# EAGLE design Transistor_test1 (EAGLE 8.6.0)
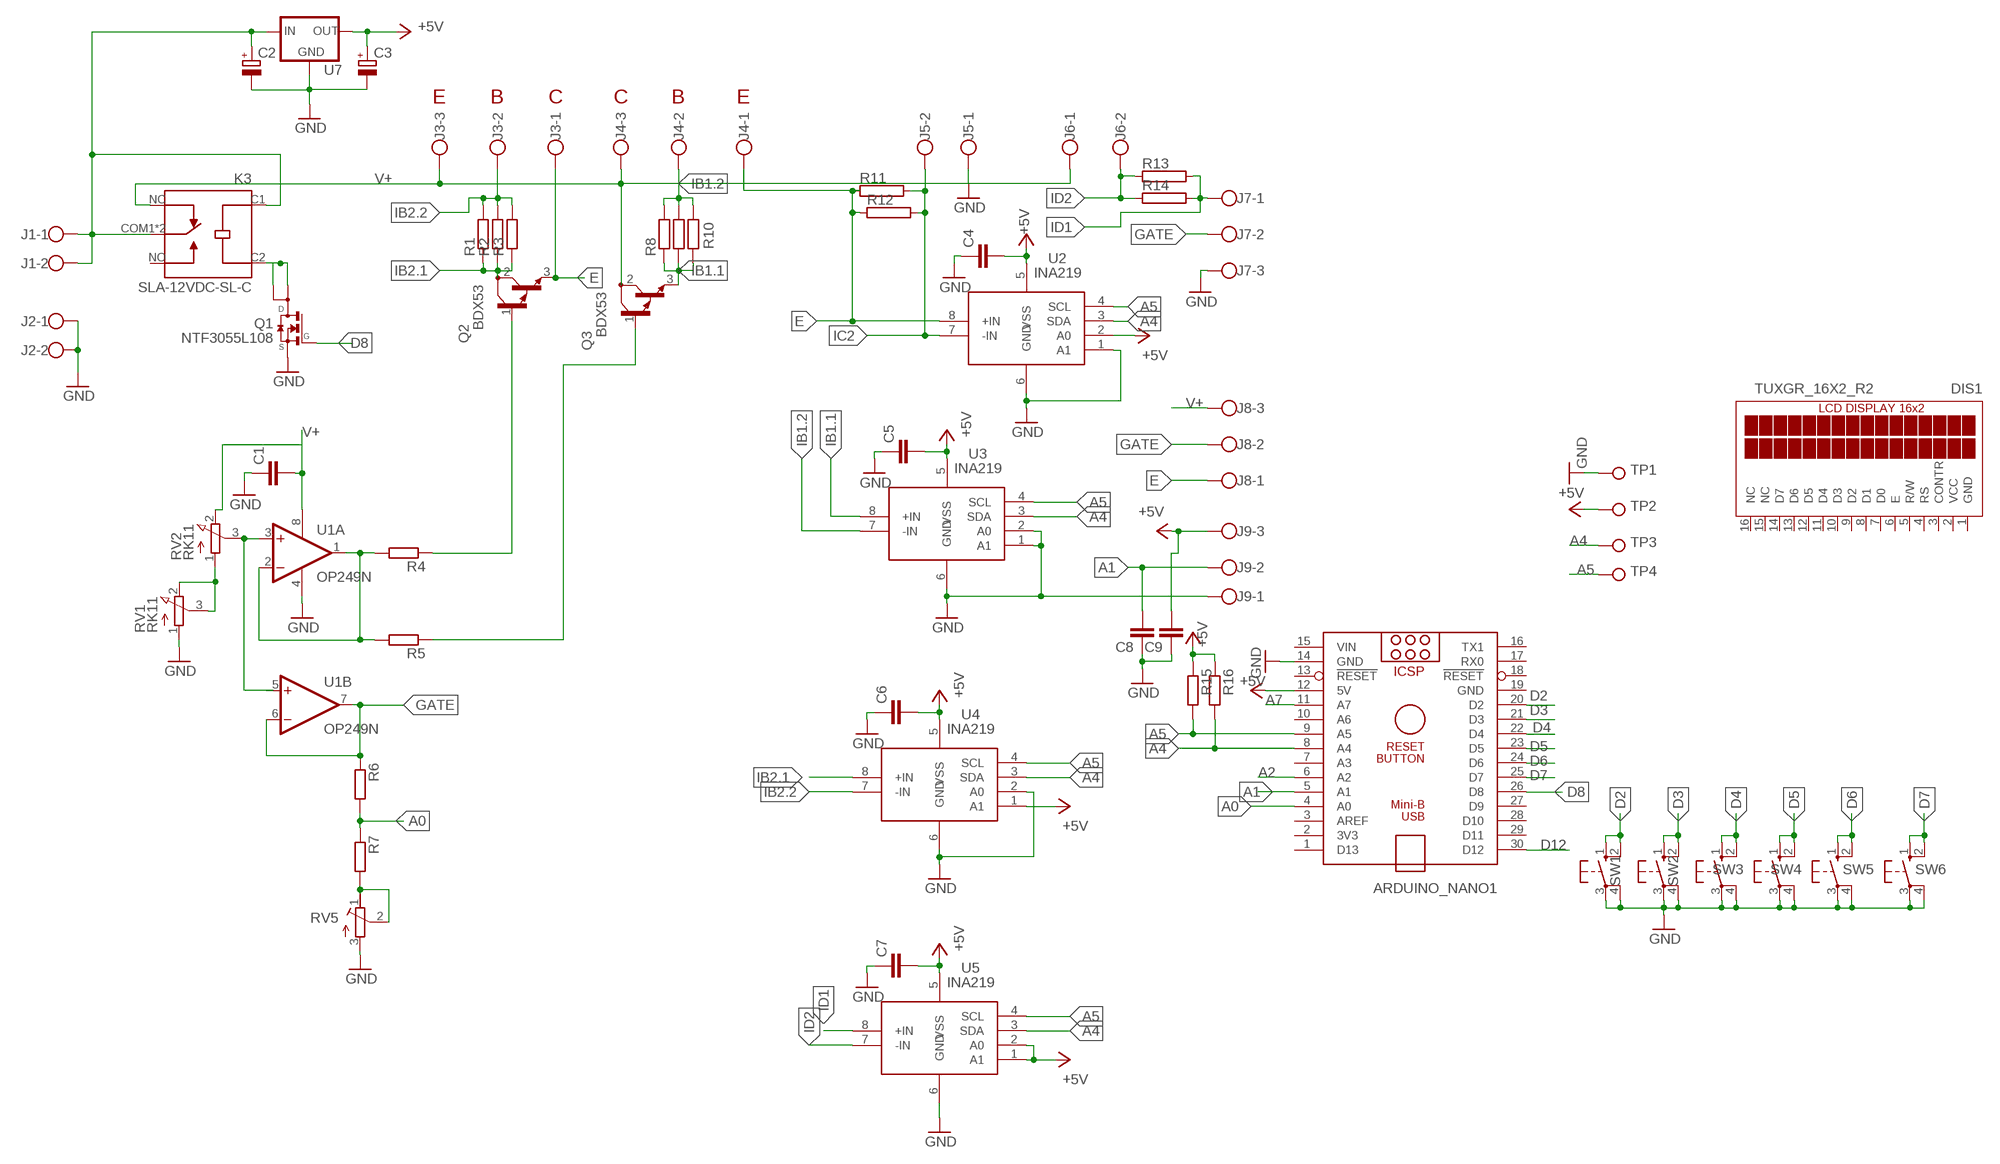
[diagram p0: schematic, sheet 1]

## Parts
ARDUINO_NANO1  ARDUINO_NANO  [ARDUINO_NANO]
C1  C-EUC1206  [C1206]
C2  CPOL-EUE2.5-7  [E2,5-7]
C3  CPOL-EUE2.5-7  [E2,5-7]
C4  C-EUC1206  [C1206]
C5  C-EUC1206  [C1206]
C6  C-EUC1206  [C1206]
C7  C-EUC1206  [C1206]
C8  C-EUC1206  [C1206]
C9  C-EUC1206  [C1206]
DIS1  TUXGR_16X2_R2  [TUXGR_16X2_R2]
J1  W237-102  [W237-102]
J2  W237-102  [W237-102]
J3  W237-103  [W237-103]
J4  W237-103  [W237-103]
J5  W237-102  [W237-102]
J6  W237-102  [W237-102]
J7  W237-103  [W237-103]
J8  W237-103  [W237-103]
J9  W237-103  [W237-103]
K3  SLA-12VDC-SL-C  [RELAY_SLA-12VDC-SL-C]
Q1  NTF3055L108  [SOT223]
Q2  BDX53  [TO220]
Q3  BDX53  [TO220]
R1  R-EU_R2512  [R2512]
R2  R-EU_R2512  [R2512]
R3  R-EU_R2512  [R2512]
R4  R-EU_R1206  [R1206]
R5  R-EU_R1206  [R1206]
R6  R-EU_R1206  [R1206]
R7  R-EU_R1206  [R1206]
R8  R-EU_R2512  [R2512]
R9  R-EU_R2512  [R2512]
R10  R-EU_R2512  [R2512]
R11  RAC07  [AC07]
R12  RAC07  [AC07]
R13  RAC07  [AC07]
R14  RAC07  [AC07]
R15  R-EU_R1206  [R1206]
R16  R-EU_R1206  [R1206]
RV1  RK11  PTV111  [PTV111]
RV2  RK11  PTV111  [PTV111]
RV5  R-TRIMM-3386-F  [R-TRIMM-3386F]
SW1  40-XX  [B3F-40XX]
SW2  40-XX  [B3F-40XX]
SW3  40-XX  [B3F-40XX]
SW4  40-XX  [B3F-40XX]
SW5  40-XX  [B3F-40XX]
SW6  40-XX  [B3F-40XX]
TP1  TPPAD1-13Y  [P1-13Y]
TP2  TPPAD1-13Y  [P1-13Y]
TP3  TPPAD1-13Y  [P1-13Y]
TP4  TPPAD1-13Y  [P1-13Y]
U1  OP249N  [DIL08]
U2  INA219  [SO08]
U3  INA219  [SO08]
U4  INA219  [SO08]
U5  INA219  [SO08]
U7  78MXXS  [78MXXS]

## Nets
+5V: ARDUINO_NANO1.12(5V) C3.+ C4.2 C5.2 C6.2 C7.2 C9.2 J9.3 R15.1 R16.1 TP2.TP U2.2(A0) U2.5(VSS) U3.5(VSS) U4.1(A1) U4.5(VSS) U5.1(A1) U5.2(A0) U5.5(VSS) U7.OUT
+15V: C2.+ J1.1 J1.2 K3.C1(COIL1) K3.COM1(COM) K3.COM2(COM) U7.IN
A0: ARDUINO_NANO1.4(A0) R6.2 R7.1
A1: ARDUINO_NANO1.5(A1) C8.2 J9.2
A2: ARDUINO_NANO1.6(A2)
A4: ARDUINO_NANO1.8(A4) R16.2 TP3.TP U2.3(SDA) U3.3(SDA) U4.3(SDA) U5.3(SDA)
A5: ARDUINO_NANO1.9(A5) R15.2 TP4.TP U2.4(SCL) U3.4(SCL) U4.4(SCL) U5.4(SCL)
A7: ARDUINO_NANO1.11(A7)
D2: ARDUINO_NANO1.20(D2) SW1.1(S) SW1.2(S1)
D3: ARDUINO_NANO1.21(D3) SW2.1(S) SW2.2(S1)
D4: ARDUINO_NANO1.22(D4) SW3.1(S) SW3.2(S1)
D5: ARDUINO_NANO1.23(D5) SW4.1(S) SW4.2(S1)
D6: ARDUINO_NANO1.24(D6) SW5.1(S) SW5.2(S1)
D7: ARDUINO_NANO1.25(D7) SW6.1(S) SW6.2(S1)
D8: ARDUINO_NANO1.26(D8) Q1.1(G)
D12: ARDUINO_NANO1.30(D12)
E: J3.1 J4.1 J8.1 Q2.3(E) R11.1 R12.1 U2.8(+IN)
GATE: J7.2 J8.2 R6.1 U1.6(B:-IN) U1.7(B:OUT)
GND: ARDUINO_NANO1.14(GND) C1.1 C2.- C3.- C4.1 C5.1 C6.1 C7.1 C8.1 C9.1 J2.1 J2.2 J5.1 J7.3 J9.1 Q1.3(S) RV1.1(A) RV5.3(E) SW1.3(P) SW1.4(P1) SW2.3(P) SW2.4(P1) SW3.3(P) SW3.4(P1) SW4.3(P) SW4.4(P1) SW5.3(P) SW5.4(P1) SW6.3(P) SW6.4(P1) TP1.TP U1.4(P:V-) U2.1(A1) U2.6(GND) U3.1(A1) U3.2(A0) U3.6(GND) U4.2(A0) U4.6(GND) U5.6(GND) U7.GND
IB1.1: Q3.3(E) R8.1 R9.1 R10.1 U3.8(+IN)
IB1.2: J4.2 R8.2 R9.2 R10.2 U3.7(-IN)
IB2.1: Q2.2(C) R1.1 R2.1 R3.1 U4.8(+IN)
IB2.2: J3.2 R1.2 R2.2 R3.2 U4.7(-IN)
IC2: J5.2 R11.2 R12.2 U2.7(-IN)
ID1: J7.1 R13.2 R14.2 U5.8(+IN)
ID2: J6.2 R13.1 R14.1 U5.7(-IN)
N$1: Q3.1(B) R5.1
N$2: R4.2 R5.2 U1.1(A:OUT) U1.2(A:-IN)
N$4: K3.C2(COIL2) Q1.2(D) Q1.4(D2)
N$5: RV1.2(E) RV1.3(S) RV2.1(A)
N$6: R7.2 RV5.1(A) RV5.2(S)
N$7: Q2.1(B) R4.1
N$11: RV2.3(S) U1.3(A:+IN) U1.5(B:+IN)
V+: C1.2 J3.3 J4.3 J6.1 J8.3 K3.NC Q3.2(C) RV2.2(E) U1.8(P:V+)
Unconnected: ARDUINO_NANO1.1(D13) ARDUINO_NANO1.2(3V3) ARDUINO_NANO1.3(AREF) ARDUINO_NANO1.7(A3) ARDUINO_NANO1.10(A6) ARDUINO_NANO1.13(!RESET) ARDUINO_NANO1.16(TX1) ARDUINO_NANO1.17(RX0) ARDUINO_NANO1.18(!RESET) ARDUINO_NANO1.27(D9) ARDUINO_NANO1.28(D10) ARDUINO_NANO1.29(D11) DIS1.3(CONTR) DIS1.4(RS) DIS1.5(R/W) DIS1.6(E) DIS1.7(D0) DIS1.8(D1) DIS1.9(D2) DIS1.10(D3) DIS1.11(D4) DIS1.12(D5) DIS1.13(D6) DIS1.14(D7) DIS1.15(NC) DIS1.16(NC) K3.NO

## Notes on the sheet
- E | B | C | C | B | E

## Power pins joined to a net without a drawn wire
GND: ARDUINO_NANO1.19(GND) DIS1.1(GND)
VCC: DIS1.2(VCC)
VIN: ARDUINO_NANO1.15(VIN)

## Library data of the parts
ARDUINO_NANO1 = ArduinoNanoV30:ARDUINO_NANO: Arduino Nano V3.0 Overview: The Arduino Nano is a small, complete, and breadboard-friendly board based on the ATmega328 (Arduino Nano 3.x) or ATmega168 (Arduino Nano 2.x). It has more or less the same functionality of the Arduino Duemilanove, but in a different package. It lacks only a DC power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
C1 C4-C9 = rcl:C-EU: CAPACITOR, European symbol
C2 C3 = rcl:CPOL-EU: POLARIZED CAPACITOR, European symbol
DIS1 = display-lcd:TUXGR_16X2_R2: Tuxgraphics LCD display 16x2 characters reflective, without background light Source: tuxgr_12x2_r2.pdf; OC_FARNELL: unknown; OC_NEWARK: unknown
J1 J2 J5 J6 = con-wago-500:W237-102: WAGO SCREW CLAMP; MPN: 237-102; OC_FARNELL: unknown; OC_NEWARK: 70K9898
J3 J4 J7-J9 = con-wago-500:W237-103: WAGO SCREW CLAMP; MPN: 237-103; OC_FARNELL: unknown; OC_NEWARK: 18M7116
K3 = SLA-12VDC-SL-C:SLA-12VDC-SL-C: SUBMINATURE HIGH POWER RELAY Check availability; AVAILABILITY: Not in stock; CHECK_PRICES: https://www.snapeda.com/parts/SLA-12VDC-SL-C/Songle+Relay/view-part/?ref=eda; DESCRIPTION: SUBMINATURE HIGH POWER RELAY; MF: Songle Relay; MP: SLA-12VDC-SL-C; PACKAGE: None; PRICE: None; SNAPEDA_LINK: https://www.snapeda.com/parts/SLA-12VDC-SL-C/Songle+Relay/view-part/?ref=snap
Q1 = NTF3055L108:NTF3055L108: N-Channel MOSFET 3.0 A, 60 V Check availability; AVAILABILITY: In Stock; CHECK_PRICES: https://www.snapeda.com/parts/NTF3055L108/Onsemi/view-part/?ref=eda; DESCRIPTION: N-Channel 60 V 3A (Ta) 1.3W (Ta) Surface Mount SOT-223 (TO-261); MF: ON Semiconductor; MP: NTF3055L108; PACKAGE: TO-261-4 ON Semiconductor; PRICE: None; PURCHASE-URL: https://www.snapeda.com/api/url_track_click_mouser/?unipart_id=2731930&manufacturer=ON Semiconductor&part_name=NTF3055L108&search_term=ntf3055; SNAPEDA_LINK: https://www.snapeda.com/parts/NTF3055L108/Onsemi/view-part/?ref=snap
Q2 Q3 = transistor:BDX53: NPN BIPOLAR DARLINGTON TRANSISTOR
R1-R3 R8-R10 = resistor:R-EU_: RESISTOR, European symbol
R4-R7 R15 R16 = rcl:R-EU_: RESISTOR, European symbol
R11-R14 = resistor-power:R: Power Resitor; OC_FARNELL: unknown; OC_NEWARK: unknown
RV1 RV2 = pot:PTV111
RV5 = rcl:R-TRIMM-3386-F
SW1-SW6 = switch-omron:40-XX: OMRON SWITCH; MF: OMRON COMPONENTS USA; MPN: B3F-4000; OC_FARNELL: 176434; OC_NEWARK: 36K3105
TP1-TP4 = testpad:TP: Test pad
U1 = linear:OP249: Dual, Precision JFET High Speed Operational Amplifier Source: http://www.analog.com/static/imported-files/data_sheets/OP249.pdf
U2-U5 = burr-brown:INA219: Bidirectional Current/Power Monitor With I2C Interface
U7 = v-reg:78MXXS: VOLTAGE REGULATOR

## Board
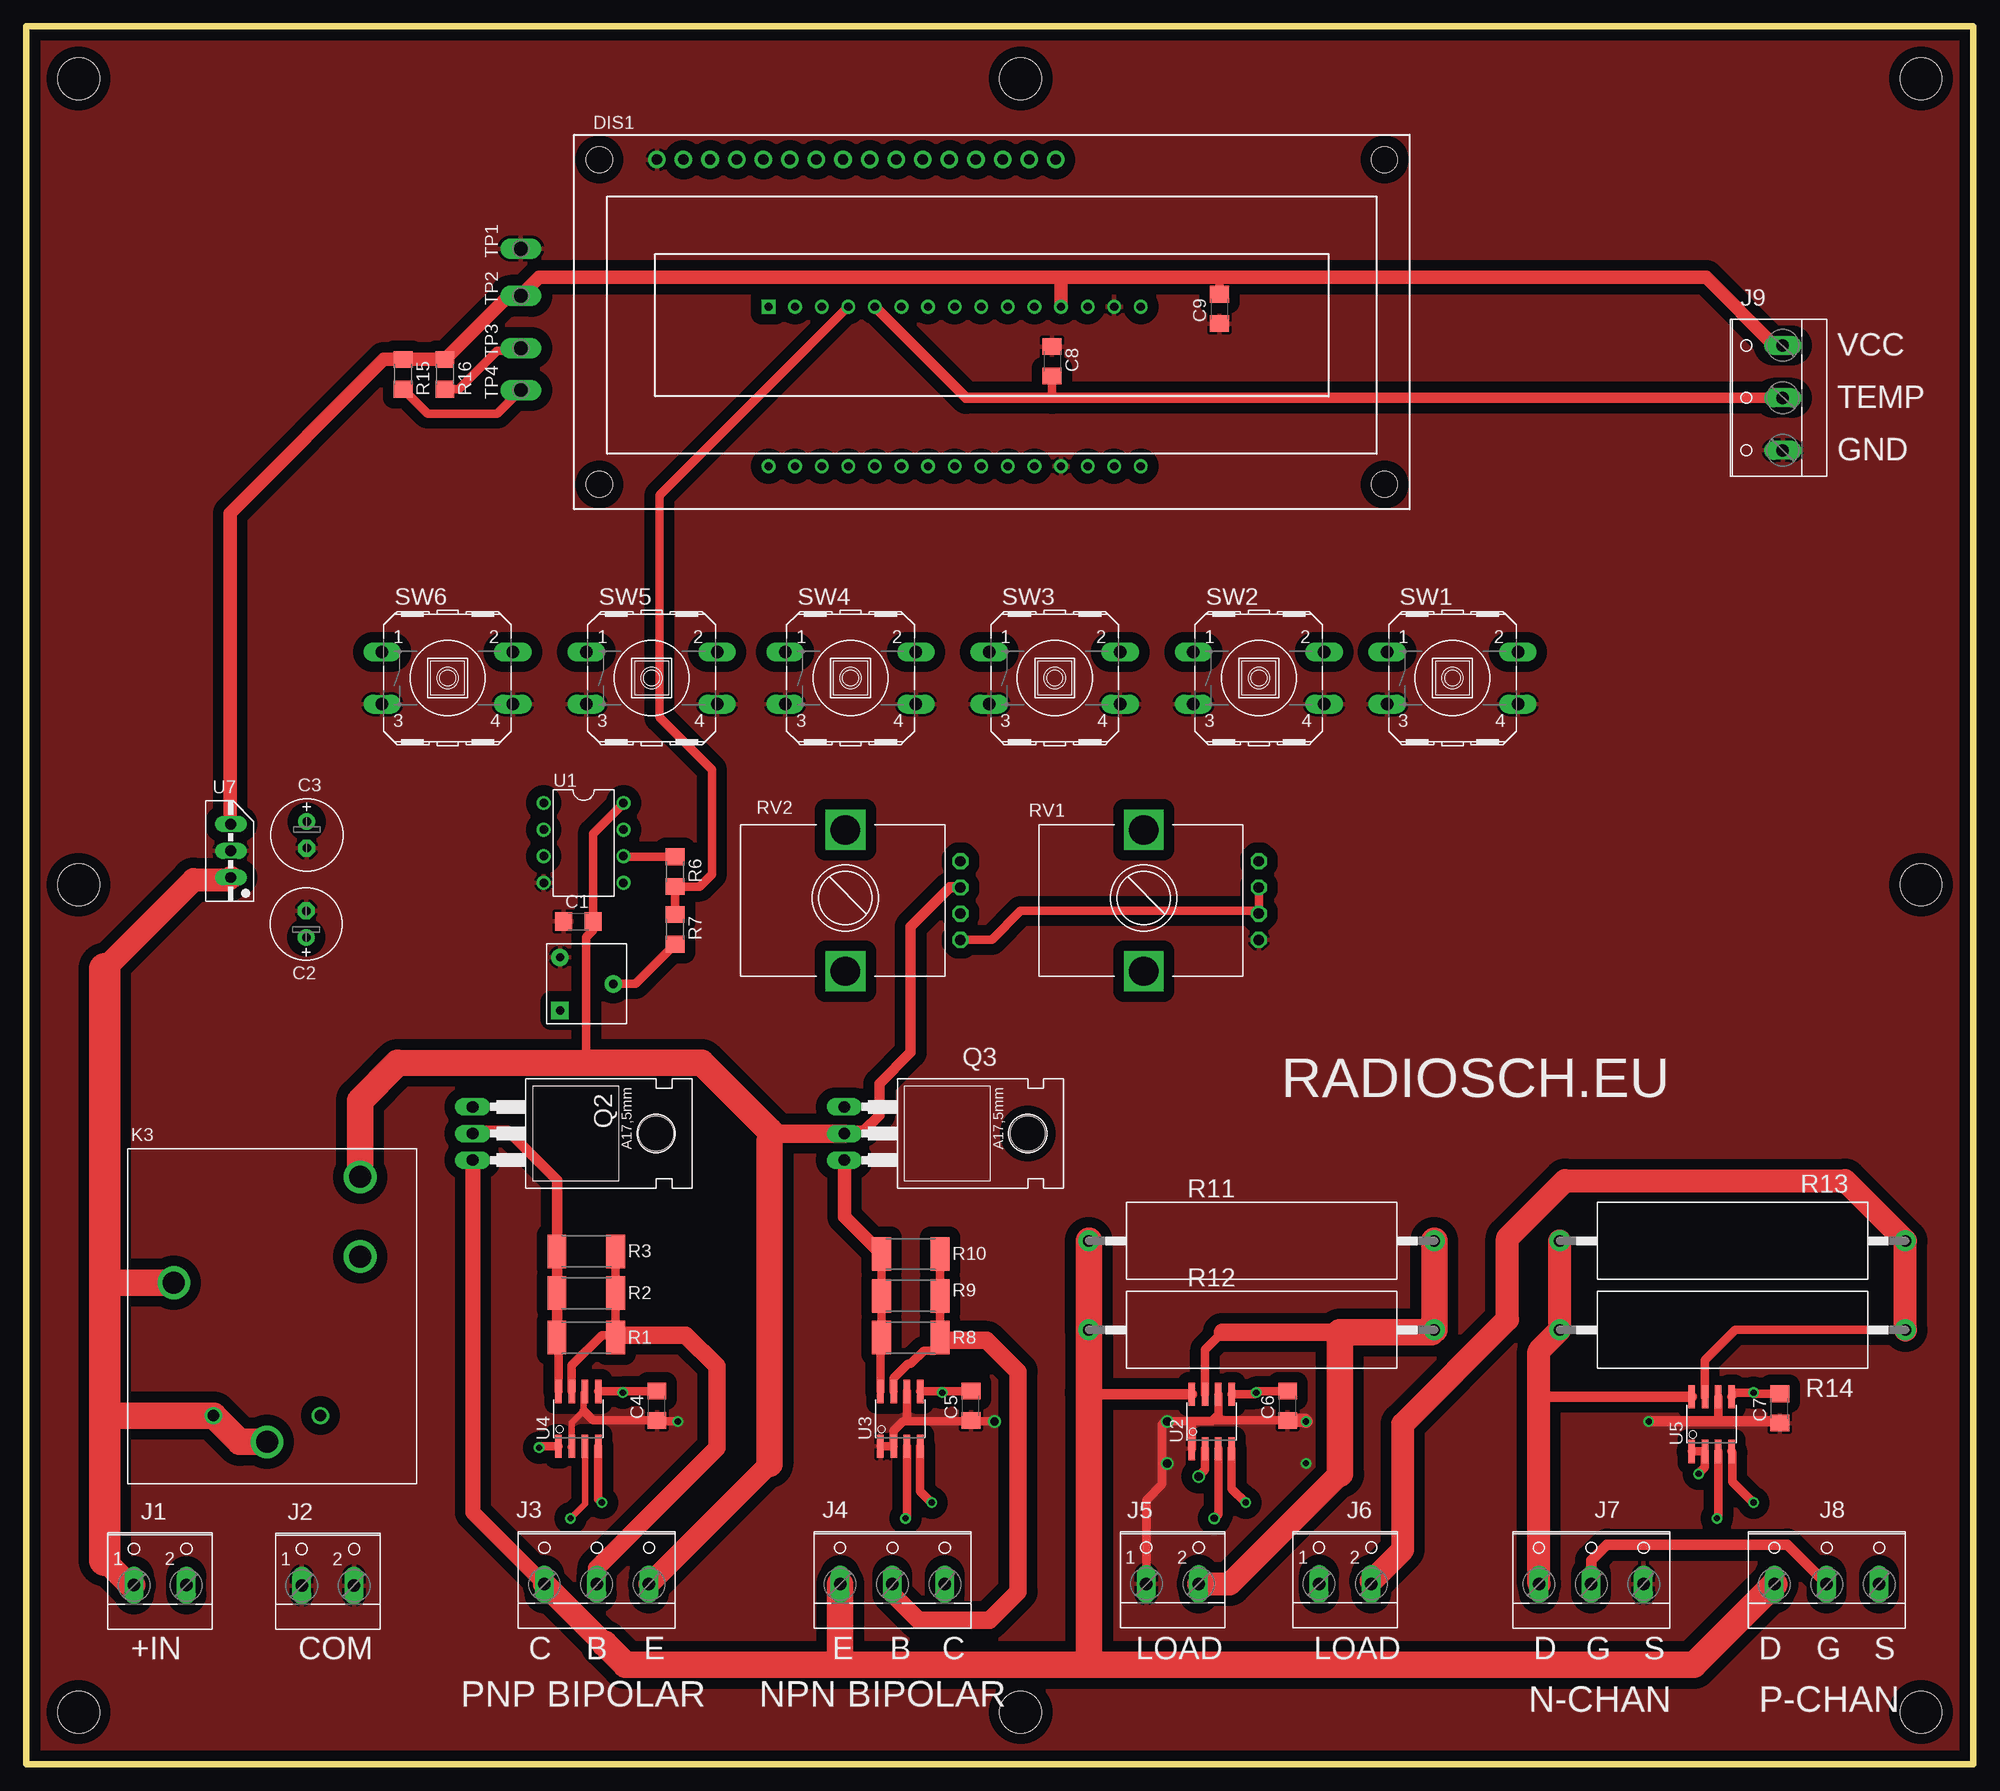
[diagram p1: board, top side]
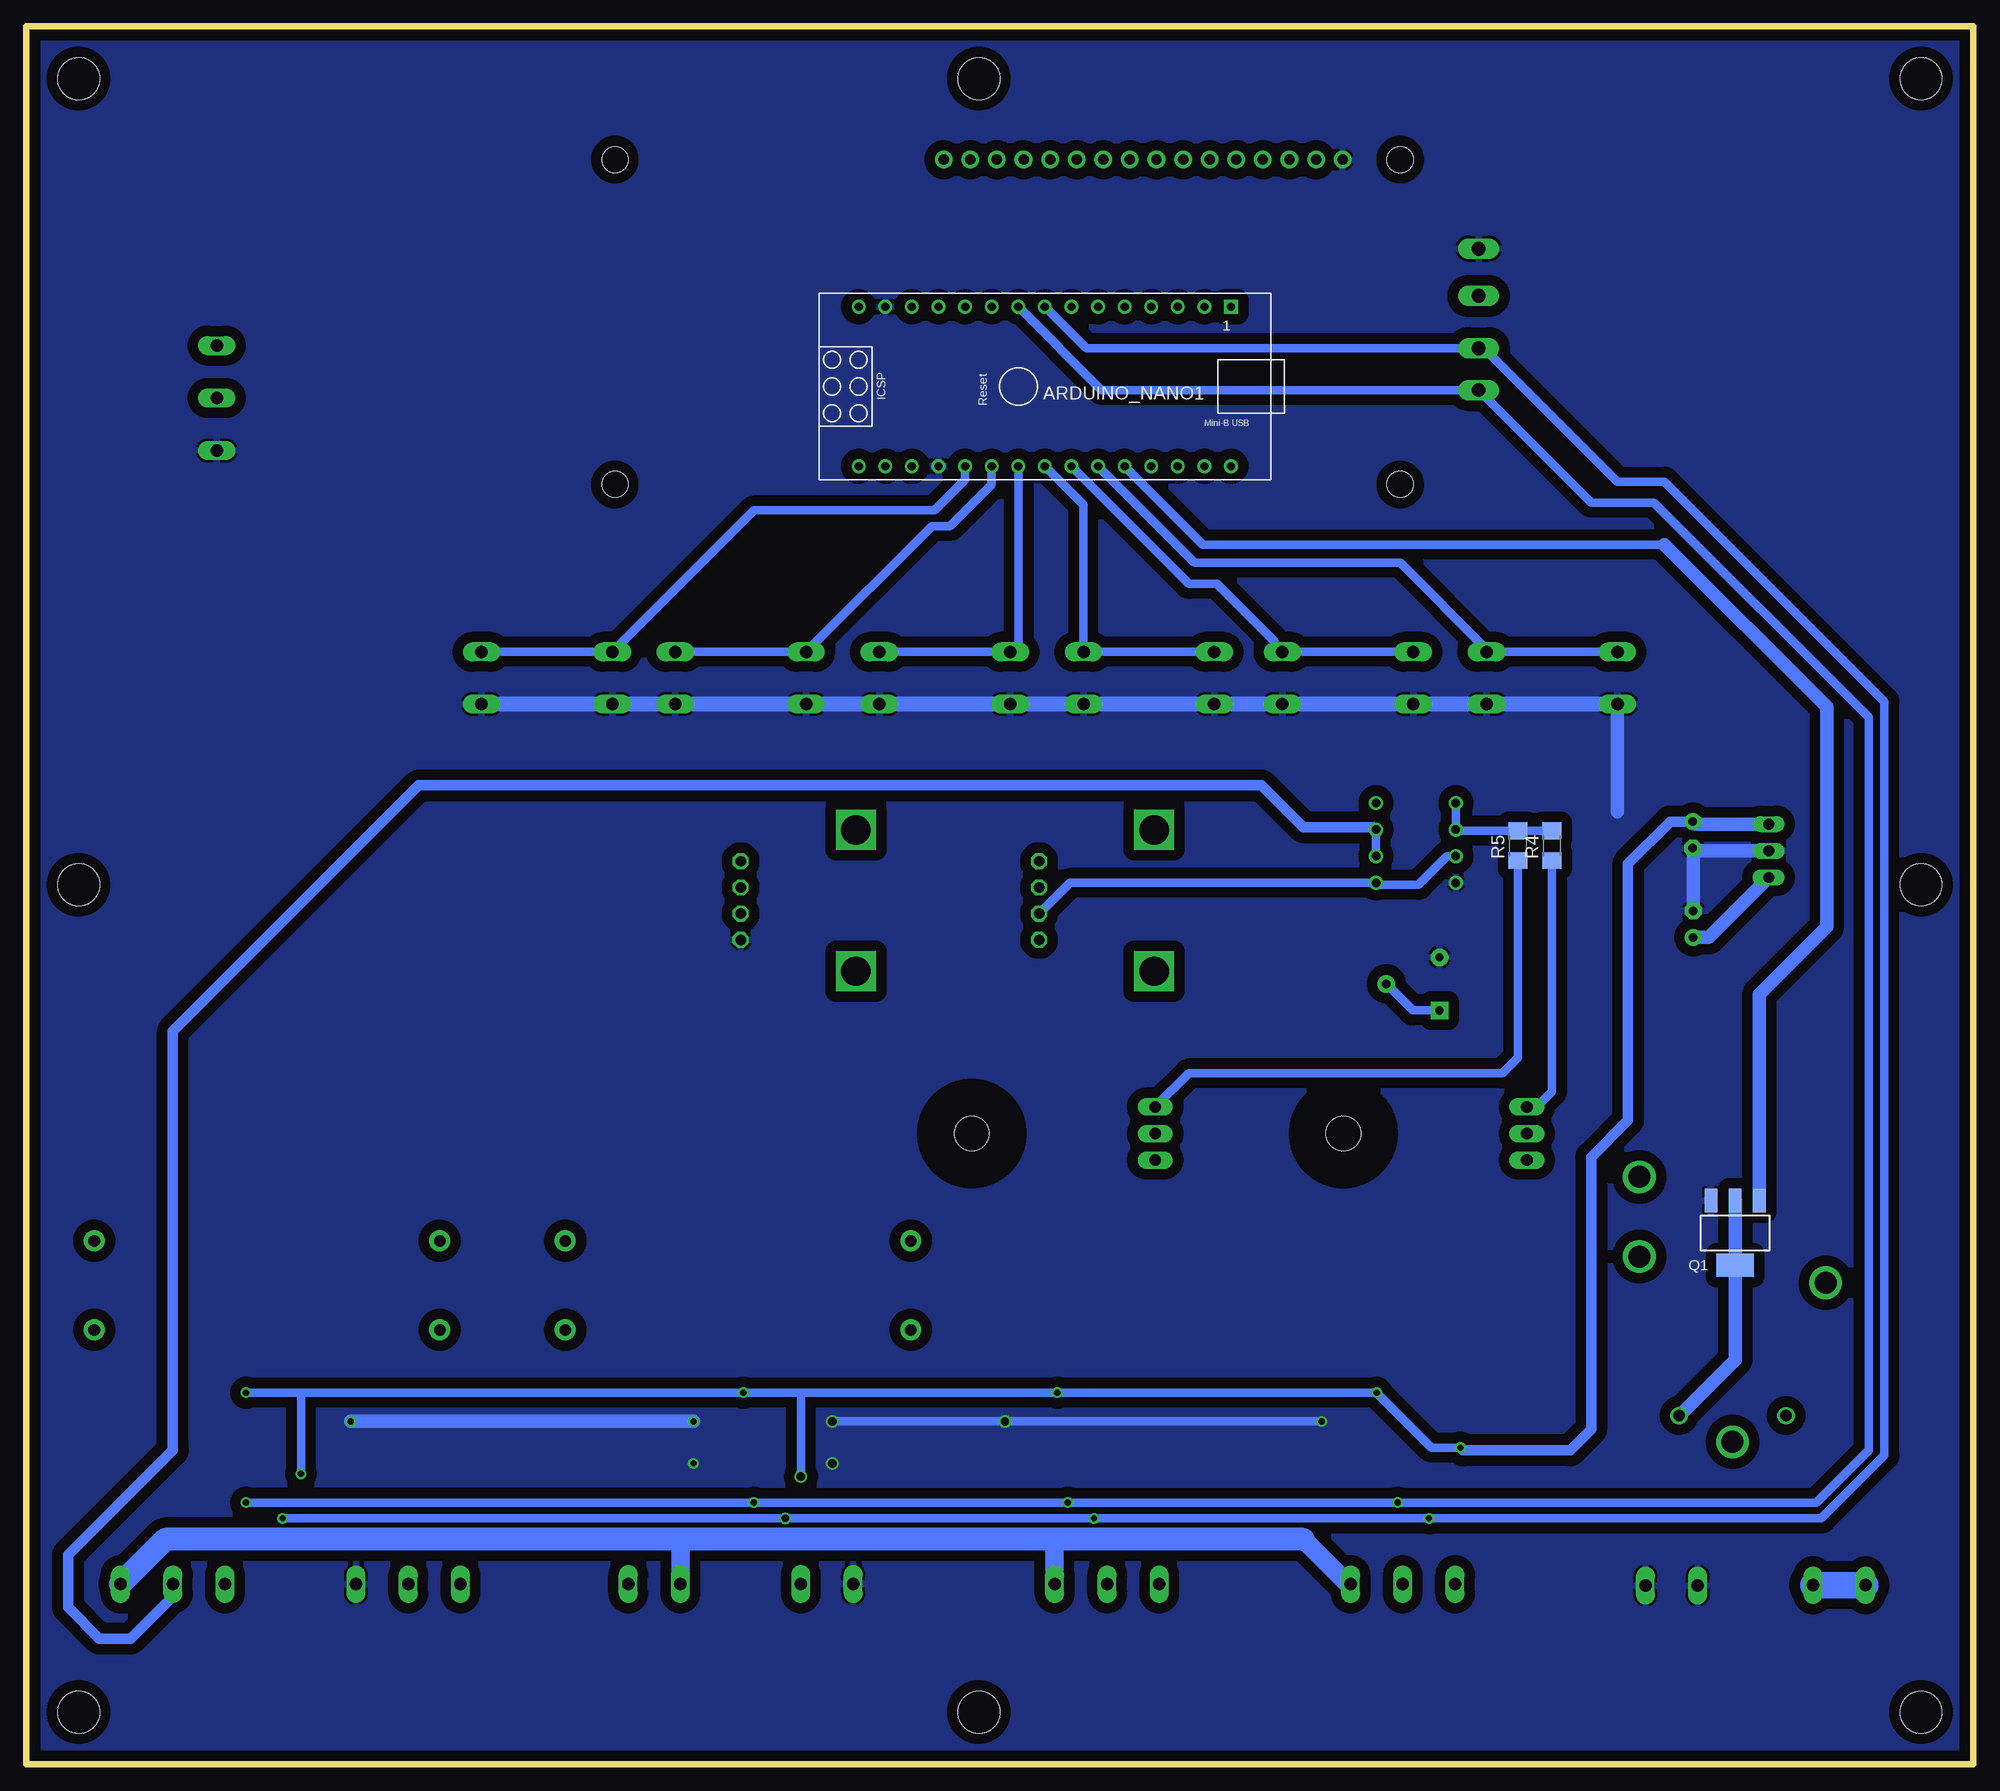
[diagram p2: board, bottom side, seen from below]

Size 186 x 166 mm. Coordinates in mm from the lower left corner, seen from the top.
Outline: 0,0 0,166 186,166 186,0 0,0
Copper layers (1*16): Top 0.035mm / dielectric 1.5mm / Bottom 0.035mm
Design rules "default *": minimum track width 10mil, minimum drill 8mil, track to track 8mil, track to pad 8mil, pad to pad 8mil, via to via 8mil, smd to smd 8mil, copper to edge 40mil, drill to drill 8mil, minimum pad ring 10mil, minimum via ring 8mil, stop-mask expansion 4mil, vias tented up to drill 0mil, thermal gap 10mil
Holes 4 mm at 5,5 5,84 5,161 95,5 181,5 181,84 181,161 95,161

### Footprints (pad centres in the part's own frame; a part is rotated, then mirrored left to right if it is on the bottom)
ARDUINO_NANO = drill 0.8 square: 1 -20.32,-7.62 | drill 0.8: 2 -17.78,-7.62; 3 -15.24,-7.62; 4 -12.7,-7.62; 5 -10.16,-7.62; 6 -7.62,-7.62; 7 -5.08,-7.62; 8 -2.54,-7.62; 9 0,-7.62; 10 2.54,-7.62; 11 5.08,-7.62; 12 7.62,-7.62; 13 10.16,-7.62; 14 12.7,-7.62; 15 15.24,-7.62; 16 15.24,7.62; 17 12.7,7.62; 18 10.16,7.62; 19 7.62,7.62; 20 5.08,7.62; 21 2.54,7.62; 22 0,7.62; 23 -2.54,7.62; 24 -5.08,7.62; 25 -7.62,7.62; 26 -10.16,7.62; 27 -12.7,7.62; 28 -15.24,7.62; 29 -17.78,7.62; 30 -20.32,7.62
C1206 = smd 1.6 x 1.8: 1 -1.4,0; 2 1.4,0
E2,5-7 = drill 0.813 pad 1.6: + -1.27,0 | drill 0.813 pad 1.6 octagon: - 1.27,0
TUXGR_16X2_R2 = drill 1 pad 1.676: 1 -32,15.5; 2 -29.46,15.5; 3 -26.92,15.5; 4 -24.38,15.5; 5 -21.84,15.5; 6 -19.3,15.5; 7 -16.76,15.5; 8 -14.22,15.5; 9 -11.68,15.5; 10 -9.14,15.5; 11 -6.6,15.5; 12 -4.06,15.5; 13 -1.52,15.5; 14 1.02,15.5; 15 3.56,15.5; 16 6.1,15.5 | hole 2.5: -37.5,-15.5; 37.5,-15.5; -37.5,15.5; 37.5,15.5
W237-102 = drill 1.194 long: 1 -2.5,-1.27; 2 2.5,-1.27
W237-103 = drill 1.194 long: 1 -5,-1.29; 2 0,-1.29; 3 5,-1.29
RELAY_SLA-12VDC-SL-C = drill 1.1: C1 -5.1,-15.2; C2 5.1,-15.2 | drill 2.1: COM1 0,-17.7; COM2 -8.9,-2.5; NC 8.9,7.6; NO 8.9,0
SOT223 = smd 1.219 x 2.235: 1 -2.311,-3.099; 2 0,-3.099; 3 2.311,-3.099 | smd 3.6 x 2.2: 4 0,3.099
TO220 = drill 1.118 long: 1 -2.54,-6.35; 2 0,-6.35; 3 2.54,-6.35 | hole 3.302: 0,11.176
R2512 = smd 1.8 x 3.2: 1 -2.8,0; 2 2.8,0
R1206 = smd 1.6 x 1.803: 1 -1.422,0; 2 1.422,0
AC07 = drill 1.1 pad 2: 1 -16.5,0; 2 16.5,0
PTV111 = drill 1 octagon: 1 3,-11; 2 8,-11; 3 5.5,-11; 4 10.5,-11 | drill 2.8 square: P$1 0,0; P$2 13.5,0
R-TRIMM-3386F = drill 0.8 pad 1.676 square: 1 0,0 | drill 0.8 pad 1.676: 2 5.08,2.54; 3 0,5.08
B3F-40XX = drill 1.194 long: 1 -6.248,2.489; 2 6.248,2.489; 3 -6.248,-2.489; 4 6.248,-2.489
P1-13Y = drill 1.321 pad 1.905 long: TP 0,0
DIL08 = drill 0.813 pad 1.27: 1 -3.81,-3.81; 2 -1.27,-3.81; 3 1.27,-3.81; 4 3.81,-3.81; 5 3.81,3.81; 6 1.27,3.81; 7 -1.27,3.81; 8 -3.81,3.81
SO08 = smd 0.61 x 2.21: 1 -1.905,-2.616; 2 -0.635,-2.616; 3 0.635,-2.616; 4 1.905,-2.616; 5 1.905,2.616; 6 0.635,2.616; 7 -0.635,2.616; 8 -1.905,2.616
78MXXS = drill 1.016 long: GND 0,-2.54; IN -2.54,-2.54; OUT 2.54,-2.54

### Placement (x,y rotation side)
ARDUINO_NANO1  91.23,131.59 180 bottom
C1  52.75,80.5 0 top
C2  26.75,80.25 90 top
C3  26.8,88.77 270 top
C4  60.25,34.25 90 top
C5  90.25,34.25 90 top
C6  120.5,34.25 90 top
C7  167.5,34 90 top
C8  98,134 270 top
C9  114,139 90 top
DIS1  92.25,137.75 0 top
J1  12.8,18.38 0 top
J2  28.82,18.35 0 top
J3  54.5,18.5 0 top
J4  82.75,18.5 0 top
J5  109.5,18.5 0 top
J6  126,18.5 0 top
J7  149.5,18.5 0 top
J8  172,18.5 0 top
J9  166.5,130.5 90 top
K3  23,48.5 0 top
Q1  22.75,50.75 180 bottom
Q2  49,60.25 270 top
Q3  84.5,60.25 270 top
R1  53.5,40.75 0 top
R2  53.5,45 0 top
R3  53.5,49 0 top
R4  40.25,87.75 90 bottom
R5  43.5,87.75 90 bottom
R6  62,85.25 270 top
R7  62,79.75 270 top
R8  84.5,40.75 0 top
R9  84.5,44.75 0 top
R10  84.5,48.75 0 top
R11  118,50 0 top
R12  118,41.5 0 top
R13  163,50 180 top
R14  163,41.5 180 top
R15  36,132.75 270 top
R16  40,132.75 270 top
RV1  106.75,75.75 90 top
RV2  78.25,75.75 90 top
RV5  51,72 0 top
SW1  136.25,103.75 0 top
SW2  117.75,103.75 0 top
SW3  98.25,103.75 0 top
SW4  78.75,103.75 0 top
SW5  59.75,103.75 0 top
SW6  40.25,103.75 0 top
TP1  47.25,144.75 90 top
TP2  47.25,140.25 90 top
TP3  47.25,135.25 90 top
TP4  47.25,131.25 90 top
U1  53.25,88 270 top
U2  113.25,32.75 0 top
U3  83.5,33 0 top
U4  52.75,33 0 top
U5  161,32.5 0 top
U7  17,87.25 90 top

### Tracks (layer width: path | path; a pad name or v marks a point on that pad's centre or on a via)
+5V  (via drill 0.6, 0.8)
  Top 0.813: U4.5 56.88,35.62 v57,35.5 57.15,35.65 C4.2 | U5.5 163.29,35.5 v165,35.5 165.1,35.4 C7.2 | U2.5 117.37,35.37 v117.5,35.5 117.65,35.65 C6.2 | U3.5 87.38,35.62 v87.5,35.5 87.65,35.65 C5.2 | U4.1 49.13,30.38 v49,30.25 | U2.2 112.61,28.11 v112,27.5 | U5.1 U5.2 160.37,28.36 v159.75,27.75 | C9.2 114,142
  Top 1.27: J9.3 167,135.5 160.5,142 114,142 98.5,142 | 98.5,142 49,142 TP2.TP 46.08,140.25 R16.1 R15.1 34.17,134.17 19.5,119.5 19.5,89.83 U7.OUT | ARDUINO_NANO1.12 98.85,141.65 98.5,142
  Bottom 0.813: 112.25,35.5 v87.5,35.5 v57,35.5 51.75,30.25 v49,30.25 | 112.25,35.5 v117.5,35.5 159.75,35.5 | 159.75,35.5 v165,35.5 | v112,27.5 112,35.25 112.25,35.5 | v159.75,27.75 159.75,35.5
  Bottom 1.016: C3.+ 28.96,90.04 33,86 33,61.5 36.5,58 36.5,32 38.5,30 48.75,30 v49,30.25
  Bottom 1.27: U7.OUT 26.55,89.79 C3.+
+15V
  Top 1.27: 7.8,33.3 7.5,33
  Top 2.184: 7.5,76 16,84.5 19.33,84.5 U7.IN | 7.5,19.5 10,17 10.19,17 J1.1
  Top 2.54: 7.8,33.3 K3.C1 20.4,30.8 K3.COM1 | K3.COM2 7.5,46
  Top 3: 7.5,19.5 7.5,33 7.5,46 7.5,76
  Bottom 1.27: C2.+ 25.27,78.98 U7.IN
  Bottom 2.54: J1.1 J1.2
A0
  Top 0.813: R7.1 R6.2 64.33,83.83 65.5,85 65.5,95 60.5,100 60.5,121.18 ARDUINO_NANO1.4
A1
  Top 0.813: C8.2 98,130.5
  Top 1.016: J9.2 98,130.5 89.78,130.5 ARDUINO_NANO1.5
A4  (via drill 0.6, 0.7)
  Top 0.61: U4.3 53.38,24.89 v52,23.5
  Top 0.813: R16.2 41.33,131.33 45,135 47,135 TP3.TP | U3.3 84.14,23.64 v84,23.5 | U2.3 113.89,23.89 v113.5,23.5 | U5.3 161.63,23.64 v161.5,23.5
  Bottom 0.813: v161.5,23.5 v113.5,23.5 v84,23.5 v52,23.5 14.5,23.5 8.5,29.5 8.5,101.5 29.5,122.5 34,122.5 46.75,135.25 TP3.TP 84.73,135.25 ARDUINO_NANO1.8
A5  (via drill 0.6)
  Top 0.813: U4.4 54.66,25.34 v55,25 | TP4.TP 45,129 38.33,129 R15.2 | U2.4 115.16,26.34 v116.5,25 | U3.4 85.41,26.09 v86.5,25 | v165,25 163,27 163,29.79 U5.4
  Bottom 0.813: v165,25 v116.5,25 v86.5,25 v55,25 15,25 10,30 10,100 30.5,120.5 36.5,120.5 TP4.TP 83.27,131.25 ARDUINO_NANO1.9
D2
  Bottom 0.813: ARDUINO_NANO1.20 96.31,122.69 99.25,119.75 116.49,119.75 SW1.1 SW1.2
D3
  Bottom 0.813: ARDUINO_NANO1.21 93.77,122.23 97.75,118.25 99.49,118.25 SW2.1 SW2.2
D4
  Bottom 0.813: ARDUINO_NANO1.22 91.23,107.01 SW3.1 SW3.2
D5
  Bottom 0.813: ARDUINO_NANO1.23 85,120.28 SW4.2 SW4.1
D6
  Bottom 0.813: 86.25,123.87 ARDUINO_NANO1.24 74.93,112.75 72.25,112.75 66.74,107.24 66.74,106.24 SW5.2 SW5.1
D7
  Bottom 0.813: ARDUINO_NANO1.25 74.39,114.75 54.75,114.75 46.5,106.5 SW6.2 SW6.1
D8
  Bottom 0.813: 29.5,116.5 73.6,116.5 ARDUINO_NANO1.26
  Bottom 1.27: Q1.1 20.44,73.56 14,80 14,101 29.5,116.5
E
  Top 1.016: U2.8 101.63,35.37 101.5,35.5
  Top 1.422: Q2.3 42.65,24.06 J3.1
  Top 1.676: 55.21,11.5 55.25,11.5 | 101.5,10 102,9.5 | 77.75,9.75 78,9.5
  Top 2.184: 55.21,11.5 J3.1
  Top 2.54: J8.1 159.29,9.5 102,9.5 78,9.5 57.25,9.5 55.25,11.5 | 101.5,10 101.5,35.5 R12.1 R11.1 | J4.1 77.75,9.75
GATE
  Top 0.813: R6.1 57.12,86.67 U1.6
  Top 1.016: J7.2 149.5,19.5 151,21 168.21,21 J8.2
  Bottom 0.813: U1.6 U1.7
  Bottom 1.016: U1.7 57.29,89.5 64,89.5 68,93.5 148.5,93.5 172,70 172,30 182,20 182,15 179,12 176,12 172,16 J8.2
GND  (via drill 0.6, 0.8)
  Top 0.61: 52,30.27 U4.2 52.12,32.62 53.25,33.75 53.25,35.48 U4.6
  Top 0.813: 84,32.75 83.75,32.75 82.86,31.86 U3.2 U3.1 | 84,32.75 90.35,32.75 | 90.35,32.75 90.85,32.75 | 90.85,32.75 C5.1 90.35,32.75 | U3.6 84.14,32.88 84,32.75 | v62.25,32.75 60.35,32.75 C4.1 54.15,32.85 53.25,33.75 | U2.6 113.89,33.38 113.35,32.85 | 111.5,32.75 113.25,32.75 113.35,32.85 | 111.5,32.75 v109,32.75 108.75,32.75 108.5,32.5 108.5,26.75 107,25.25 J5.1 | U2.1 111.34,32.59 111.5,32.75 | C6.1 113.35,32.85 | 90.85,32.75 v92.5,32.75 | U5.6 161.63,32.88 161.5,32.75
  Top 1.016: v155,32.75 161.5,32.75 167.35,32.75 C7.1
  Top 1.27: C6.1 122.15,32.85 v122.25,32.75
  Bottom 0.813: v109,32.75 v92.5,32.75 v62.25,32.75
  Bottom 1.27: U7.GND 26.55,87.25 C3.- 26.75,87.45 C2.- | 34,91 34,100.76 34.5,101.26 | v122.25,32.75 v155,32.75
  Bottom 1.422: SW6.3 34.5,101.26 SW6.4 52.74,101.26 52.75,101.25 SW5.3 SW5.4 SW4.3 SW4.4 SW3.3 SW3.4 SW2.3 SW2.4 SW1.3 SW1.4
  other vias: 109,28.75 122.25,28.75
  pour Bottom (isolate 1.016): 1,165 185,165 185,1.5 1,1.5
  pour Top (isolate 1.016): 1.5,164.5 184.5,164.5 184.5,1 1.5,1
IB1.1
  Top 0.813: U3.8 81.59,40.65 R8.1 R9.1 R10.1
  Top 1.27: Q3.3 78.15,52.3 R10.1
IB1.2
  Top 0.813: U3.7 82.86,36.87 84.25,38.25 84.5,38.25 85.75,39.5 86.75,39.5 87.25,40 87.25,40.7 R8.2 R9.2 R10.2
  Top 1.676: J4.2 82.75,16.25 85.25,13.75 92,13.75 94.75,16.5 94.75,37.5 91.75,40.5 87.55,40.5 R8.2
IB2.1
  Top 0.813: U4.8 50.84,40.6
  Top 1.016: 50.84,40.6 R1.1 R2.1 R3.1 50.7,55.8 46,60.5 42.9,60.5 Q2.2
IB2.2
  Top 0.813: U4.7 52.12,38.12 55,41 56.05,41 R1.2 R2.2 R3.2
  Top 1.676: J3.2 54.5,18.75 66,30.25 66,38 63,41 56.55,41 R1.2
IC2
  Top 0.813: U2.7 112.61,39.62 114.25,41.25
  Top 1.016: 134.25,41.25 R12.2
  Top 1.676: 114.25,41.25 125.5,41.25
  Top 2.184: J5.2 114.98,17.23 125.5,27.75
  Top 2.54: 134.25,41.25 125.5,41.25 125.5,27.75 | R12.2 R11.2
ID1
  Top 1.016: U5.8 144.63,35.12 144.5,35.25
  Top 2.184: R13.2 R14.2 144.5,39.5 144.5,35.25 J7.1
ID2
  Top 0.813: U5.7 160.37,38.62 163.25,41.5 R14.1
  Top 1.676: J6.2 128.5,17.5
  Top 2.184: 128.5,17.5 131.5,20.5 131.5,32.5 141.5,42.5 141.5,50.25 147,55.75 173.75,55.75 R13.1 R14.1
N$1
  Bottom 0.813: R5.1 43.5,67.5 45,66 74.94,66 Q3.1
N$2
  Bottom 0.813: R4.2 R5.2 49.34,89.17 U1.2 U1.1
N$4
  Bottom 1.27: Q1.2 Q1.4 22.75,38.65 K3.C2
N$5
  Top 0.813: RV2.1 92.25,78.75 95,81.5 117.5,81.5 RV1.3 RV1.2
N$6
  Top 0.813: RV5.2 58.21,74.54 R7.2
  Bottom 0.813: RV5.1 53.54,72 RV5.2
N$7
  Bottom 0.813: R4.1 40.25,64.25 42,62.5 42.36,62.5 Q2.1
N$11
  Bottom 0.813: U1.3 50.27,86.73 53,84 56.87,84 U1.5 86.31,84.19 RV2.3
V+
  Top 0.813: U1.8 54.15,88.9 C1.2 54.15,79.65 53.5,79 53.5,67
  Top 1.016: RV2.2 88.25,83.75 84.5,80 84.5,68 81.5,65 81.5,62 80,60.5 77.75,60.5 77.5,60.25
  Top 1.778: 71,60.5 71,59.5 71.75,60.25 77.5,60.25 Q3.2
  Top 2: 71,28.71 J3.3
  Top 2.5: 35.5,67 53.5,67
  Top 2.54: 53.5,67 64.5,67 71,60.5 | 71,59.5 71,28.71 | K3.NC 31.9,63.4 35.5,67
  Bottom 1.778: J3.3 59.71,17.21 64,21.5 | J6.1 123.5,21.5 | J4.3 87.75,21.25 88,21.5
  Bottom 2.184: 64,21.5 88,21.5 123.5,21.5 172.71,21.5 J8.3

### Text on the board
tPlace: VCC | TEMP | GND | RADIOSCH.EU | +IN | COM | C | B | E | E | B | C | LOAD | LOAD | D | G | S | D | G | S | PNP BIPOLAR | NPN BIPOLAR | N-CHAN | P-CHAN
